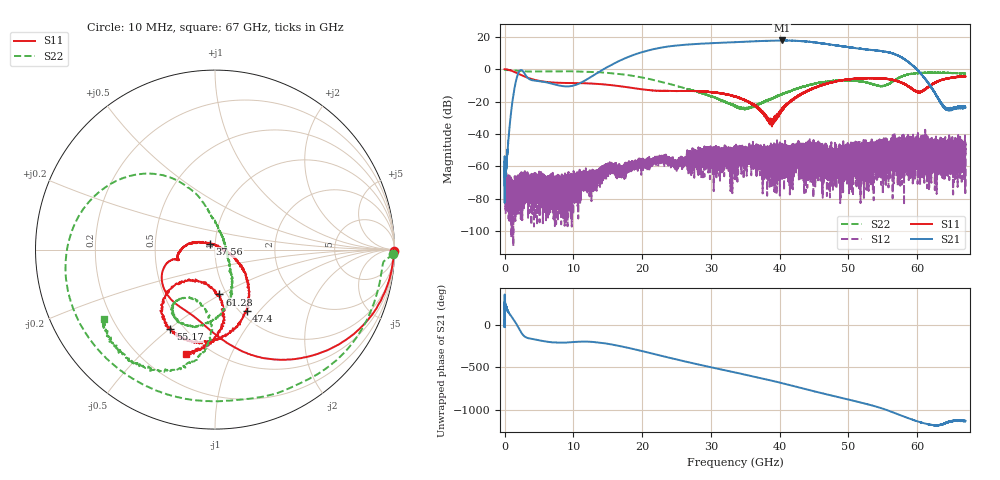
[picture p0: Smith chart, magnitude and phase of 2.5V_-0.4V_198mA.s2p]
! MARKI MICROWAVE INC.
! Date:  10/21/2020
! Model Number:  AMM-7210CH
! Description:  2-port Small Signal S-parameter data for AMM-7210CH
! Frequency Range:  10 MHz to 67 GHz
! Port Configuration:  PORT 1: Input
!  PORT 2: Output
! Bias Condition: Vd = +2.5V, Vg = -0.4V
! AMM-7210CH s2p files are only valid for small signal conditions (below -10 dBm input power)
# Hz S  dB  R 50
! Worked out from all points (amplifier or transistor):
!   20001 points, 10 MHz to 67 GHz, reference 50 ohm
!   highest |S21| = 17.7 dB at 40.29 GHz (marker M1)
!   |S21| within 3 dB of that: 25.31 GHz to 48.03 GHz (22.72 GHz wide, 61.9 % of centre)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
!   unconditionally stable (mu >= 1): start of sweep to end of sweep
!   at 11.17 GHz: K = 1547.41, MAG = -2.1 dB, |S12| = -73.7 dB
!   at 33.51 GHz: K = 28.01, MAG = 16.8 dB, |S12| = -51.9 dB
!   at 67 GHz: K = 884.52, MAG = -18.3 dB, |S12| = -51.9 dB
!   S11 on the Smith chart (normalised r, x): 10 MHz: open; 37.56 GHz: 0.94, +0.06; 47.4 GHz: 1.07, -0.86; 55.17 GHz: 0.42, -0.50; 61.28 GHz: 0.92, -0.49; 67 GHz: 0.38, -0.68
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1e7  -0.02 -0.5  -56.92 -24.6  -60.85 -64.1  -0.05 -1.5
2.21732e9  -3.21 -62.3  -0.92 -62.2  -71.71 56.1  -1.13 -61.4
1.117723e10  -8.66 -133.2  -8.20 162.0  -72.36 149.1  -1.46 -169.4
1.700201e10  -10.65 -162.0  5.71 105.9  -64.34 150.7  -3.16 149.2
1.988928e10  -12.37 -166.8  10.35 53.1  -56.59 116.6  -5.06 130.7
2.234112e10  -13.35 -164.8  12.93 4.8  -55.92 111.8  -7.38 117.6
2.475276e10  -13.48 -164.8  14.46 -42.4  -57.83 74.4  -10.00 107.7
2.786779e10  -13.46 -169.8  15.52 -100.6  -51.16 109.8  -13.74 98.1
3.097613e10  -14.53 178.5  16.19 -155.7  -55.40 37.1  -18.43 81.0
3.3505e10  -16.87 166.4  16.66 160.3  -51.85 35.1  -23.03 50.6
3.578601e10  -21.19 153.8  17.07 120.1  -54.34 -15.9  -23.59 -10.1
3.756124e10  -27.25 133.1  17.40 87.7  -49.40 -60.2  -20.58 -37.7
4.029444e10  -24.83 -8.1  17.70 35.5  -48.93 -70.0  -15.41 -57.3
4.237783e10  -17.32 -28.0  17.50 -6.6  -53.98 175.6  -12.15 -68.2
4.467223e10  -12.30 -42.8  16.75 -53.8  -51.99 120.5  -9.49 -81.4
4.739873e10  -8.27 -62.8  15.13 -107.8  -57.82 109.1  -7.46 -99.4
5.103293e10  -5.98 -90.8  12.94 -178.0  -54.41 60.1  -7.10 -121.3
5.516622e10  -5.88 -119.3  10.95 90.0  -46.88 176.0  -10.33 -107.7
5.583612e10  -6.20 -123.9  10.37 71.3  -59.33 143.8  -9.14 -97.6
5.868319e10  -10.52 -137.8  4.54 -16.3  -46.59 -152.4  -3.32 -106.2
6.12824e10  -12.01 -84.5  -6.77 -82.1  -51.40 -176.0  -2.19 -124.5
6.7e10  -4.50 -106.2  -23.59 -48.2  -51.94 -79.0  -2.66 -147.9
